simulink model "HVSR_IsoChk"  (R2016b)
settings: Solver=VariableStepAuto  StartTime=0.0  StopTime=10.0  RelTol=1e-3
undefined symbols (not defined in the file or in its folder): bin2dec, enmActv, enmBmsMode, enmCctErr, enmSWSta, HVSR_bIsoResShieldCal, HVSR_bSw1EnaByMnl_C, HVSR_bSw2EnaByMnl_C, HVSR_bSw3EnaByMnl_C, HVSR_bSwEnaByMnl_C, HVSR_bVldEnaByMnl_C, HVSR_cntIsoChkCnfDiag_C, HVSR_cntIsoChkCnfLv1Diag_C, HVSR_cntIsoChkDiag_CW, HVSR_cntPwrDown_C, HVSR_cofPosVoltfilter_C, HVSR_cofResGain_C, HVSR_deltInsRes_C, HVSR_InsResCtrlSw_C, HVSR_kSlopeVal_C, HVSR_numBgnTimeCnt_C, HVSR_numCycleTimeCnt_C, HVSR_numIsoCnst_C, HVSR_numSlopeCnfrm_C, HVSR_ResFirstCtrlSw_C, HVSR_resIsoFaultLvl1Thres_C, HVSR_resIsoFaultLvl2Thres_C, HVSR_ResR1_C, HVSR_ResR2_C, HVSR_ResR3_C, HVSR_resRstnUpLim_C, HVSR_rIsoCnfHysDiag_C, HVSR_rIsoCnfHysLv1Diag_C, HVSR_stBMSModeLvl_C, HVSR_tiChkFilteTime_C, HVSR_tiIsoChkCycl_T, HVSR_tiIsoChkDebounce_C, HVSR_tiIsoVldChkDebounce_C, HVSR_tiTaskTime_C, HVSR_tiVoltDiffThres_C, HVSR_uBattVoltRngHi_C, HVSR_uBattVoltRngLo_C, HVSR_uIsoKVoltThres_C, HVSR_uIsoPosVoltFilter_C, HVSR_uIsoVoltThres_C
libraries: simulink x78
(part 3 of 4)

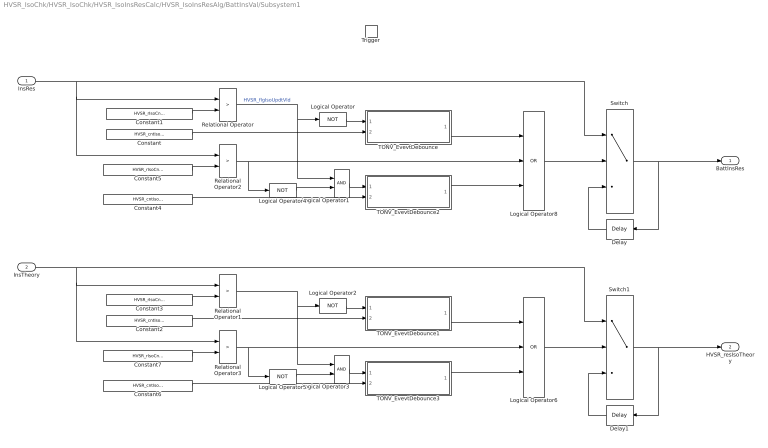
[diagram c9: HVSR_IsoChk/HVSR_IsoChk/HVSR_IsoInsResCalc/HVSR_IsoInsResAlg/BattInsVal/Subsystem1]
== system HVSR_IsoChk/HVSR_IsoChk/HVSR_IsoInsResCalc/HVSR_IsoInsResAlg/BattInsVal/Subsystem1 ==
  InsRes : Inport
  InsTheory : Inport  Port=2
  Trigger : TriggerPort  TriggerType=falling  VariantControl=Variant  PortDimensions=1
  Constant : Constant  Value=HVSR_cntIsoChkCnfDiag_C
  Constant1 : Constant  Value=HVSR_rIsoCnfHysDiag_C
  Constant2 : Constant  Value=HVSR_cntIsoChkCnfDiag_C
  Constant3 : Constant  Value=HVSR_rIsoCnfHysDiag_C
  Constant4 : Constant  Value=HVSR_cntIsoChkCnfLv1Diag_C
  Constant5 : Constant  Value=HVSR_rIsoCnfHysLv1Diag_C
  Constant6 : Constant  Value=HVSR_cntIsoChkCnfLv1Diag_C
  Constant7 : Constant  Value=HVSR_rIsoCnfHysLv1Diag_C
  Delay : Delay  DelayLength=1  InitialCondition=0
  Delay1 : Delay  DelayLength=1  InitialCondition=0
  Logical Operator{,2,4..5} (4 alike) : Logic  Operator=NOT  AllPortsSameDT=off  OutDataTypeStr=boolean
  Logical Operator1 : Logic  AllPortsSameDT=off  OutDataTypeStr=boolean
  Logical Operator3 : Logic  AllPortsSameDT=off  OutDataTypeStr=boolean
  Logical Operator6 : Logic  Operator=OR  Inputs=3  AllPortsSameDT=off  OutDataTypeStr=boolean
  Logical Operator8 : Logic  Operator=OR  Inputs=3  AllPortsSameDT=off  OutDataTypeStr=boolean
  Relational Operator{,1..3} (4 alike) : RelationalOperator  Operator=>  OutDataTypeStr=boolean  RndMeth=Simplest
  Switch : Switch  Criteria=u2 > Threshold
  Switch1 : Switch  Criteria=u2 > Threshold
  TONV_EvevtDebounce : Subsystem  TreatAsAtomicUnit=on  RTWFcnName=TONV_EvevtDebounce  RTWFileName=SrvLib
  TONV_EvevtDebounce1 : Subsystem  TreatAsAtomicUnit=on  RTWFcnName=TONV_EvevtDebounce  RTWFileName=SrvLib
  TONV_EvevtDebounce2 : Subsystem  TreatAsAtomicUnit=on  RTWFcnName=TONV_EvevtDebounce  RTWFileName=SrvLib
  TONV_EvevtDebounce3 : Subsystem  TreatAsAtomicUnit=on  RTWFcnName=TONV_EvevtDebounce  RTWFileName=SrvLib
  BattInsRes : Outport
  HVSR_resIsoTheory : Outport  Port=2
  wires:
  Constant1/1 -> Relational Operator/2
  InsRes/1 -> Relational Operator2/1, Relational Operator/1, Switch/1
  Relational Operator/1 -> Logical Operator1/1, Logical Operator/1  "HVSR_flgIsoUpdtVld"
  Switch/1 -> Delay/1, BattInsRes/1
  Logical Operator/1 -> TONV_EvevtDebounce/1(u)
  Constant/1 -> TONV_EvevtDebounce/2(T)
  Delay/1 -> Switch/3
  Constant5/1 -> Relational Operator2/2
  Logical Operator4/1 -> Logical Operator1/2
  Constant4/1 -> TONV_EvevtDebounce2/2(T)
  Relational Operator2/1 -> Logical Operator8/2, Logical Operator4/1
  TONV_EvevtDebounce2/1(y) -> Logical Operator8/3
  TONV_EvevtDebounce/1(y) -> Logical Operator8/1
  Logical Operator1/1 -> TONV_EvevtDebounce2/1(u)
  Logical Operator8/1 -> Switch/2
  Constant3/1 -> Relational Operator1/2
  InsTheory/1 -> Relational Operator3/1, Relational Operator1/1, Switch1/1
  Relational Operator1/1 -> Logical Operator3/1, Logical Operator2/1
  Switch1/1 -> HVSR_resIsoTheory/1, Delay1/1
  Logical Operator2/1 -> TONV_EvevtDebounce1/1(u)
  Constant2/1 -> TONV_EvevtDebounce1/2(T)
  Delay1/1 -> Switch1/3
  Constant7/1 -> Relational Operator3/2
  Logical Operator5/1 -> Logical Operator3/2
  Constant6/1 -> TONV_EvevtDebounce3/2(T)
  Relational Operator3/1 -> Logical Operator6/2, Logical Operator5/1
  TONV_EvevtDebounce3/1(y) -> Logical Operator6/3
  TONV_EvevtDebounce1/1(y) -> Logical Operator6/1
  Logical Operator3/1 -> TONV_EvevtDebounce3/1(u)
  Logical Operator6/1 -> Switch1/2

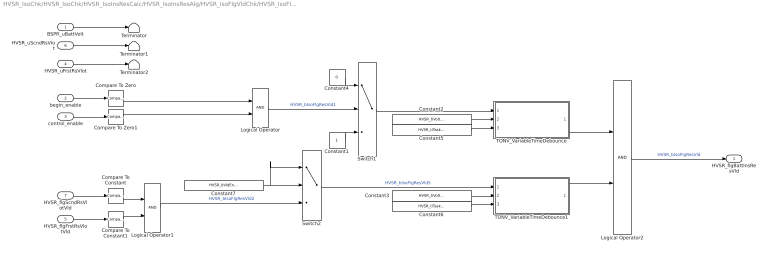
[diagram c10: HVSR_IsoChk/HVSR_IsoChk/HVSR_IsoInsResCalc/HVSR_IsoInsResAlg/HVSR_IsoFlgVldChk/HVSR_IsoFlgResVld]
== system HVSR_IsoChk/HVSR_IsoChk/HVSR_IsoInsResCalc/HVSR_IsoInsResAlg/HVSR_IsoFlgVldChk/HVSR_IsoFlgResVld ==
  BSPR_uBattVolt : Inport
  begin_enable : Inport  Port=2
  control_enable : Inport  Port=3
  HVSR_uFrstRsVlot : Inport  Port=4
  HVSR_flgFrstRsVlotVld : Inport  Port=5
  HVSR_uScndRsVlot : Inport  Port=6
  HVSR_flgScndRsVlotVld : Inport  Port=7
  Compare To Constant : simulink/Logic and Bit Operations/Compare To Constant  relop===  const=1  OutDataTypeStr=boolean
  Compare To Constant1 : simulink/Logic and Bit Operations/Compare To Constant  relop===  const=1  OutDataTypeStr=boolean
  Compare To Zero : simulink/Logic and Bit Operations/Compare To Zero  relop===  OutDataTypeStr=boolean
  Compare To Zero1 : simulink/Logic and Bit Operations/Compare To Zero  relop===  OutDataTypeStr=boolean
  Constant1 : Constant  OutDataTypeStr=boolean
  Constant2 : Constant  Value=HVSR_tiVoltDiffThres_C
  Constant3 : Constant  Value=HVSR_tiVoltDiffThres_C
  Constant4 : Constant  Value=0  OutDataTypeStr=boolean
  Constant5 : Constant  Value=HVSR_tiTaskTime_C
  Constant6 : Constant  Value=HVSR_tiTaskTime_C
  Constant7 : Constant  Value=HVSR_bVldEnaByMnl_C
  Logical Operator : Logic  AllPortsSameDT=off  OutDataTypeStr=boolean
  Logical Operator1 : Logic  AllPortsSameDT=off  OutDataTypeStr=boolean
  Logical Operator2 : Logic  AllPortsSameDT=off  OutDataTypeStr=boolean
  Switch1 : Switch  Criteria=u2 > Threshold
  Switch2 : Switch  Criteria=u2 ~= 0
  TONV_VariableTimeDebounce : Subsystem  TreatAsAtomicUnit=on  RTWFcnName=TONV_VariableTimeDebounce  RTWFileName=SrvLib
  TONV_VariableTimeDebounce1 : Subsystem  TreatAsAtomicUnit=on  RTWFcnName=TONV_VariableTimeDebounce  RTWFileName=SrvLib
  Terminator : Terminator
  Terminator1 : Terminator
  Terminator2 : Terminator
  HVSR_flgBattInsResVld : Outport
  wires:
  Constant4/1 -> Switch1/1
  Logical Operator/1 -> Switch1/2  "HVSR_bIsoFlgResVld1"
  Compare To Zero1/1 -> Logical Operator/2
  Compare To Zero/1 -> Logical Operator/1
  control_enable/1 -> Compare To Zero1/1
  begin_enable/1 -> Compare To Zero/1
  Logical Operator2/1 -> HVSR_flgBattInsResVld/1  "HVSR_bIsoFlgResVld"
  Constant3/1 -> TONV_VariableTimeDebounce1/2(T)
  Constant6/1 -> TONV_VariableTimeDebounce1/3(dT)
  TONV_VariableTimeDebounce1/1(y) -> Logical Operator2/2
  Constant2/1 -> TONV_VariableTimeDebounce/2(T)
  Constant5/1 -> TONV_VariableTimeDebounce/3(dT)
  Switch1/1 -> TONV_VariableTimeDebounce/1(u)
  TONV_VariableTimeDebounce/1(y) -> Logical Operator2/1
  BSPR_uBattVolt/1 -> Terminator/1
  HVSR_uScndRsVlot/1 -> Terminator1/1
  HVSR_uFrstRsVlot/1 -> Terminator2/1
  HVSR_flgScndRsVlotVld/1 -> Compare To Constant/1
  HVSR_flgFrstRsVlotVld/1 -> Compare To Constant1/1
  Logical Operator1/1 -> Switch2/3  "HVSR_bIsoFlgResVld2"
  Constant1/1 -> Switch1/3
  Constant7/1 -> Switch2/1, Switch2/2
  Switch2/1 -> TONV_VariableTimeDebounce1/1(u)  "HVSR_bIsoFlgResVld5"
  Compare To Constant/1 -> Logical Operator1/1
  Compare To Constant1/1 -> Logical Operator1/2

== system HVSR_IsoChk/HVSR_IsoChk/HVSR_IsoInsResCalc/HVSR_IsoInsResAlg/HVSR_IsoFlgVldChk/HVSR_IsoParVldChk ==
  HVSR_flgBattInsResVld : Inport
  HVSR_uFrstRsVlot : Inport  Port=2
  HVSR_flgFrstRsVlotVld : Inport  Port=3
  HVSR_uScndRsVlot : Inport  Port=4
  HVSR_flgScndRsVlotVld : Inport  Port=5
  In6 : Inport  Port=6
  IsoSwtLastTEna : Inport  Port=7
  Compare To Zero{,1..3} (4 alike) : simulink/Logic and Bit Operations/Compare To Zero  relop=~=  OutDataTypeStr=boolean
  Constant : Constant  Value=0  OutDataTypeStr=boolean
  Logical Operator : Logic  Inputs=6  AllPortsSameDT=off  OutDataTypeStr=boolean
  Switch : Switch  Criteria=u2 ~= 0
  HVSR_flgInsResVld : Outport
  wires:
  Switch/1 -> HVSR_flgInsResVld/1
  Compare To Zero3/1 -> Logical Operator/4
  Compare To Zero2/1 -> Logical Operator/3
  Compare To Zero1/1 -> Logical Operator/2
  Compare To Zero/1 -> Logical Operator/1
  HVSR_flgBattInsResVld/1 -> Switch/1
  Constant/1 -> Switch/3
  Logical Operator/1 -> Switch/2  "HVSR_bIsoFlgResVld3"
  IsoSwtLastTEna/1 -> Logical Operator/6
  HVSR_uScndRsVlot/1 -> Compare To Zero2/1
  HVSR_flgScndRsVlotVld/1 -> Compare To Zero3/1
  HVSR_uFrstRsVlot/1 -> Compare To Zero/1
  HVSR_flgFrstRsVlotVld/1 -> Compare To Zero1/1
  In6/1 -> Logical Operator/5

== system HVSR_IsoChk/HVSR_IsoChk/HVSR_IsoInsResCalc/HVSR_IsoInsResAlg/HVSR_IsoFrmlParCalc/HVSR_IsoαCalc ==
  HVSR_uIsoRsVolt : Inport  OutDataTypeStr=single
  HVSR_kSlopeVal : Inport  Port=2  OutDataTypeStr=single
  HVSR_tiIsoChkCycl_T : Inport  Port=3  OutDataTypeStr=single
  HVSR_numSlopeCnfrm : Inport  Port=4
  BSPR_uBattVolt : Inport  Port=5
  Action Port : ActionPort  InitializeStates=reset  ActionType=then
  HVSR_IsoαParCalc : Subsystem
  HVSR_uRsFrstSlopeFilter : Subsystem
  HVSR_uRsVoltFilter : Subsystem
  Logical Operator : Logic  AllPortsSameDT=off  OutDataTypeStr=boolean
  Terminator : Terminator
  HVSR_uIsoFrstRsVolt : Outport  InitialOutput=0
  HVSR_uFrstRsVlot : Outport  Port=2  InitialOutput=0
  HVSR_flgFrstRsVlotVld : Outport  Port=3
  HVSR_numIsoFrstVal : Outport  Port=4
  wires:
  HVSR_uRsVoltFilter/1(HVSR_uIsoFrstRsVolt) -> HVSR_uIsoFrstRsVolt/1
  BSPR_uBattVolt/1 -> HVSR_IsoαParCalc/2(BSPR_uBattVolt)
  HVSR_uRsVoltFilter/3(HVSR_flgFrstRsKVld) -> Logical Operator/1  "HVSR_flgFrstRsKVld"
  HVSR_IsoαParCalc/1(HVSR_numIsoFrstVal) -> HVSR_numIsoFrstVal/1
  HVSR_uIsoRsVolt/1 -> HVSR_uRsFrstSlopeFilter/1(HVSR_uIsoRsVolt), HVSR_uRsVoltFilter/1(HVSR_uIsoRsVolt)
  HVSR_uRsVoltFilter/2(HVSR_uFrstRsVlot) -> HVSR_uFrstRsVlot/1, [HVSR_uFrstRsVlot]
  Logical Operator/1 -> HVSR_flgFrstRsVlotVld/1, HVSR_IsoαParCalc/Trigger  "HVSR_flgFrstRsVlotVld"
  [HVSR_uFrstRsVlot] -> HVSR_IsoαParCalc/1(HVSR_uFrstRsVlot)
  HVSR_kSlopeVal/1 -> HVSR_uRsFrstSlopeFilter/2(HVSR_kSlopeVal)
  HVSR_tiIsoChkCycl_T/1 -> HVSR_uRsFrstSlopeFilter/3(HVSR_tiIsoChkCycl_T)
  HVSR_numSlopeCnfrm/1 -> HVSR_uRsFrstSlopeFilter/4(HVSR_numSlopeCnfrm)
  HVSR_uRsFrstSlopeFilter/1(HVSR_bSlopeVld) -> Logical Operator/2  "HVSR_bFrstSlopeVld"
  HVSR_uRsFrstSlopeFilter/2(ISOFilterSta) -> Terminator/1

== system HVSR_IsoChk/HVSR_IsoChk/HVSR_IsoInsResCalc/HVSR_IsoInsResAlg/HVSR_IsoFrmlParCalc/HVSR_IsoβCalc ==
  HVSR_uIsoRsVolt : Inport  OutDataTypeStr=single
  HVSR_kSlopeVal : Inport  Port=2  OutDataTypeStr=single
  HVSR_tiIsoChkCycl_T : Inport  Port=3  OutDataTypeStr=single
  HVSR_numSlopeCnfrm : Inport  Port=4  OutDataTypeStr=uint8
  BSPR_uBattVolt : Inport  Port=5
  Action Port : ActionPort  InitializeStates=reset  ActionType=elseif
  HVSR_IsoβParCalc : Subsystem
  HVSR_uRsScndSlopeFilter : Subsystem
  HVSR_uRsVoltFilter : Subsystem
  Logical Operator : Logic  AllPortsSameDT=off  OutDataTypeStr=boolean
  Terminator : Terminator
  HVSR_uIsoScndRsVolt : Outport  InitialOutput=0
  HVSR_uScndRsVlot : Outport  Port=2  InitialOutput=0
  HVSR_flgScndRsVlotVld : Outport  Port=3
  HVSR_numIsoScndVal : Outport  Port=4
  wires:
  HVSR_uRsVoltFilter/1(HVSR_uIsoScndRsVolt) -> HVSR_uIsoScndRsVolt/1
  HVSR_uIsoRsVolt/1 -> HVSR_uRsScndSlopeFilter/1(HVSR_uIsoRsVolt), HVSR_uRsVoltFilter/1(HVSR_uIsoRsVolt)
  HVSR_uRsVoltFilter/2(HVSR_uScndRsVlot) -> HVSR_uScndRsVlot/1, [HVSR_uScndRsVlot]
  BSPR_uBattVolt/1 -> HVSR_IsoβParCalc/2(BSPR_uBattVolt)
  HVSR_uRsVoltFilter/3(HVSR_flgScndRsKVld) -> Logical Operator/1  "HVSR_flgScndRsKVld"
  HVSR_IsoβParCalc/1(HVSR_numIsoScndVal) -> HVSR_numIsoScndVal/1
  HVSR_kSlopeVal/1 -> HVSR_uRsScndSlopeFilter/2(HVSR_kSlopeVal)
  HVSR_tiIsoChkCycl_T/1 -> HVSR_uRsScndSlopeFilter/3(HVSR_tiIsoChkCycl_T)
  HVSR_numSlopeCnfrm/1 -> HVSR_uRsScndSlopeFilter/4(HVSR_numSlopeCnfrm)
  HVSR_uRsScndSlopeFilter/1(HVSR_bSlopeVld) -> Logical Operator/2  "HVSR_bScndSlopeVld"
  HVSR_uRsScndSlopeFilter/2(ISOFilterSta) -> Terminator/1
  Logical Operator/1 -> HVSR_flgScndRsVlotVld/1, HVSR_IsoβParCalc/Trigger  "HVSR_flgScndRsVlotVld"
  [HVSR_uScndRsVlot] -> HVSR_IsoβParCalc/1(HVSR_uScndRsVlot)

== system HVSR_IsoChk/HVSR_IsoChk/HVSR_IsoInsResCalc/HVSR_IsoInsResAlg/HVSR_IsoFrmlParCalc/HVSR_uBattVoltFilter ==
  BSPR_uBattVolt : Inport  OutDataTypeStr=single
  Compare To Constant : simulink/Logic and Bit Operations/Compare To Constant  relop=<=  const=HVSR_uIsoVoltThres_C  OutDataTypeStr=boolean
  Constant2 : Constant  Value=0  OutDataTypeStr=single
  Subsystem2 : Subsystem
  Switch : Switch  Criteria=u2 > Threshold
  HVSR_uBattVolt : Outport
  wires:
  Constant2/1 -> Switch/3
  Switch/1 -> HVSR_uBattVolt/1
  Compare To Constant/1 -> Switch/2  "HVSR_flgBattFilterEnd"
  Subsystem2/1(Out1) -> Compare To Constant/1  "HVSR_uBattFltDiff"
  BSPR_uBattVolt/1 -> Subsystem2/1(In1), Switch/1

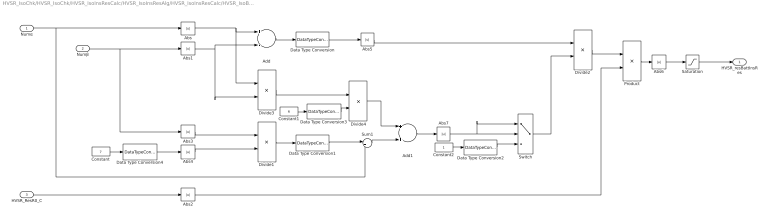
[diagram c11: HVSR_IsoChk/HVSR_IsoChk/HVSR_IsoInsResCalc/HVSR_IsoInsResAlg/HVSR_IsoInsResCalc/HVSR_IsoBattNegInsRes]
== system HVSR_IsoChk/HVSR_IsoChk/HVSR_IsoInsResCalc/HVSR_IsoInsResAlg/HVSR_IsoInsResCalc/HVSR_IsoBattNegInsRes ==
  Numα : Inport
  Numβ : Inport  Port=2
  HVSR_ResR0_C : Inport  Port=3
  Abs{,1..7} (8 alike) : Abs
  Add : Sum  Inputs=+-
  Add1 : Sum
  Constant : Constant  Value=7
  Constant1 : Constant  Value=6
  Constant2 : Constant
  Data Type Conversion : DataTypeConversion
  Data Type Conversion1 : DataTypeConversion
  Data Type Conversion2 : DataTypeConversion  OutDataTypeStr=single
  Data Type Conversion3 : DataTypeConversion  OutDataTypeStr=single
  Data Type Conversion4 : DataTypeConversion  OutDataTypeStr=single
  Divide1 : Product  Inputs=**
  Divide2 : Product  Inputs=*/
  Divide3 : Product  Inputs=**
  Divide4 : Product  Inputs=**
  Product : Product
  Saturation : Saturate  UpperLimit=60000000  LowerLimit=0
  Sum1 : Sum  Inputs=|+-
  Switch : Switch  Criteria=u2 > Threshold
  HVSR_resBattInsRes : Outport
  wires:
  Switch/1 -> Divide2/2
  Data Type Conversion2/1 -> Switch/3
  Constant2/1 -> Data Type Conversion2/1
  Divide2/1 -> Product/1
  Abs7/1 -> Switch/2, Switch/1
  Add1/1 -> Abs7/1
  Data Type Conversion/1 -> Abs5/1
  Data Type Conversion3/1 -> Divide4/2
  Constant1/1 -> Data Type Conversion3/1
  Sum1/1 -> Add1/2
  Data Type Conversion1/1 -> Sum1/1
  Data Type Conversion4/1 -> Abs4/1
  Constant/1 -> Data Type Conversion4/1
  HVSR_ResR0_C/1 -> Abs2/1
  Numβ/1 -> Abs3/1, Abs1/1
  Numα/1 -> Sum1/2, Abs/1
  Abs1/1 -> Divide3/2, Add/2
  Abs3/1 -> Divide1/1
  Abs2/1 -> Product/2
  Abs4/1 -> Divide1/2
  Abs/1 -> Divide3/1, Add/1
  Divide1/1 -> Data Type Conversion1/1
  Abs5/1 -> Divide2/1
  Add/1 -> Data Type Conversion/1
  Abs6/1 -> Saturation/1
  Product/1 -> Abs6/1
  Saturation/1 -> HVSR_resBattInsRes/1
  Divide3/1 -> Divide4/1
  Divide4/1 -> Add1/1

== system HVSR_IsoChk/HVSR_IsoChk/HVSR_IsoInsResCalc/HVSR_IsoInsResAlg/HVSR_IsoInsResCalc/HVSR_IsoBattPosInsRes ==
  Numα : Inport
  Numβ : Inport  Port=2
  HVSR_ResR0_C : Inport  Port=3
  Abs{,1..7} (8 alike) : Abs
  Add : Sum  Inputs=+-
  Add1 : Sum
  Constant : Constant  Value=7
  Constant1 : Constant  Value=6
  Constant2 : Constant
  Data Type Conversion : DataTypeConversion
  Data Type Conversion1 : DataTypeConversion
  Data Type Conversion2 : DataTypeConversion  OutDataTypeStr=single
  Data Type Conversion3 : DataTypeConversion  OutDataTypeStr=single
  Data Type Conversion4 : DataTypeConversion  OutDataTypeStr=single
  Divide1 : Product  Inputs=**
  Divide2 : Product  Inputs=*/
  Product : Product
  Saturation : Saturate  UpperLimit=60000000  LowerLimit=0
  Sum1 : Sum  Inputs=|+-
  Switch : Switch  Criteria=u2 > Threshold
  HVSR_resBattInsRes : Outport
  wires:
  Saturation/1 -> HVSR_resBattInsRes/1
  Product/1 -> Abs6/1
  Abs6/1 -> Saturation/1
  Add/1 -> Data Type Conversion/1
  Abs5/1 -> Divide2/1
  Divide1/1 -> Data Type Conversion1/1
  Abs/1 -> Add/1
  Abs4/1 -> Divide1/2
  Abs2/1 -> Product/2
  Abs3/1 -> Divide1/1
  Abs1/1 -> Add/2
  Numα/1 -> Abs/1, Sum1/2
  Numβ/1 -> Abs1/1, Abs3/1
  HVSR_ResR0_C/1 -> Abs2/1
  Constant/1 -> Data Type Conversion4/1
  Data Type Conversion4/1 -> Abs4/1
  Data Type Conversion1/1 -> Sum1/1
  Sum1/1 -> Add1/2
  Constant1/1 -> Data Type Conversion3/1
  Data Type Conversion3/1 -> Add1/1
  Data Type Conversion/1 -> Abs5/1
  Add1/1 -> Abs7/1
  Abs7/1 -> Switch/1, Switch/2
  Divide2/1 -> Product/1
  Constant2/1 -> Data Type Conversion2/1
  Data Type Conversion2/1 -> Switch/3
  Switch/1 -> Divide2/2

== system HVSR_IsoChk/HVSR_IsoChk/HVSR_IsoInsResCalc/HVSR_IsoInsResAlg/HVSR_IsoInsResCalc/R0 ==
  Constant1 : Constant  Value=HVSR_numIsoCnst_C
  Data Type Conversion1 : DataTypeConversion  OutDataTypeStr=single
  HVSR_ResR0_C : Outport
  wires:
  Constant1/1 -> Data Type Conversion1/1
  Data Type Conversion1/1 -> HVSR_ResR0_C/1

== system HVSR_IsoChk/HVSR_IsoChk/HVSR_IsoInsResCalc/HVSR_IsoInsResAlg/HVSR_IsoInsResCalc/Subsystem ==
  Rp' : Inport
  Abs : Abs
  Constant1 : Constant  Value=HVSR_ResR1_C  OutDataTypeStr=single
  Constant2 : Constant  Value=HVSR_ResR2_C  OutDataTypeStr=single
  Constant3 : Constant  Value=HVSR_ResR3_C  OutDataTypeStr=single
  Data Type Conversion : DataTypeConversion  OutDataTypeStr=single
  Data Type Conversion1 : DataTypeConversion  OutDataTypeStr=single
  Divide : Product  Inputs=/*  OutDataTypeStr=double
  Product : Product  OutDataTypeStr=double
  Saturation : Saturate  UpperLimit=60000000  LowerLimit=0
  Sum : Sum  Inputs=|++
  Sum1 : Sum  Inputs=|++
  Sum2 : Sum  Inputs=|-+
  HVSR_resIsoTheory : Outport
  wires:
  Saturation/1 -> HVSR_resIsoTheory/1
  Abs/1 -> Saturation/1
  Data Type Conversion1/1 -> Divide/2
  Product/1 -> Data Type Conversion1/1
  Data Type Conversion/1 -> Abs/1
  Divide/1 -> Data Type Conversion/1
  Sum2/1 -> Divide/1
  Rp'/1 -> Product/1, Sum2/1
  Sum1/1 -> Product/2, Sum2/2
  Constant2/1 -> Sum1/2
  Sum/1 -> Sum1/1
  Constant3/1 -> Sum/2
  Constant1/1 -> Sum/1

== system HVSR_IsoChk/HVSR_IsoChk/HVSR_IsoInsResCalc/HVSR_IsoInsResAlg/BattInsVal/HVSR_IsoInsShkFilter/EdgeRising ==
  u : Inport
  Delay1 : Delay  DelayLength=1  InitialCondition=1
  Logical Operator3 : Logic  Operator=NOT  AllPortsSameDT=off  OutDataTypeStr=boolean
  Logical Operator4 : Logic  AllPortsSameDT=off  OutDataTypeStr=boolean
  y : Outport
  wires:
  Delay1/1 -> Logical Operator3/1
  u/1 -> Logical Operator4/2, Delay1/1
  Logical Operator3/1 -> Logical Operator4/1
  Logical Operator4/1 -> y/1

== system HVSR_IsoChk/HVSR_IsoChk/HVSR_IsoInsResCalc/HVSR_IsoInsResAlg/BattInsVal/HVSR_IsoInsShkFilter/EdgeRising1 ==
  u : Inport
  Delay1 : Delay  DelayLength=1  InitialCondition=1
  Logical Operator3 : Logic  Operator=NOT  AllPortsSameDT=off  OutDataTypeStr=boolean
  Logical Operator4 : Logic  AllPortsSameDT=off  OutDataTypeStr=boolean
  y : Outport
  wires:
  Logical Operator4/1 -> y/1
  Logical Operator3/1 -> Logical Operator4/1
  u/1 -> Delay1/1, Logical Operator4/2
  Delay1/1 -> Logical Operator3/1

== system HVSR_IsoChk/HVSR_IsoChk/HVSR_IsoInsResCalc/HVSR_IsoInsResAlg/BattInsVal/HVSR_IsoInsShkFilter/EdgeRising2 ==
  u : Inport
  Delay1 : Delay  DelayLength=1  InitialCondition=1
  Logical Operator3 : Logic  Operator=NOT  AllPortsSameDT=off  OutDataTypeStr=boolean
  Logical Operator4 : Logic  AllPortsSameDT=off  OutDataTypeStr=boolean
  y : Outport
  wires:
  Delay1/1 -> Logical Operator3/1
  u/1 -> Logical Operator4/2, Delay1/1
  Logical Operator3/1 -> Logical Operator4/1
  Logical Operator4/1 -> y/1

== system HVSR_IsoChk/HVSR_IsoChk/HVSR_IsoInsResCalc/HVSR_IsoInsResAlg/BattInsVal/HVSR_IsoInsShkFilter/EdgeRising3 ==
  u : Inport
  Delay1 : Delay  DelayLength=1  InitialCondition=1
  Logical Operator3 : Logic  Operator=NOT  AllPortsSameDT=off  OutDataTypeStr=boolean
  Logical Operator4 : Logic  AllPortsSameDT=off  OutDataTypeStr=boolean
  y : Outport
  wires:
  Logical Operator4/1 -> y/1
  Logical Operator3/1 -> Logical Operator4/1
  u/1 -> Delay1/1, Logical Operator4/2
  Delay1/1 -> Logical Operator3/1

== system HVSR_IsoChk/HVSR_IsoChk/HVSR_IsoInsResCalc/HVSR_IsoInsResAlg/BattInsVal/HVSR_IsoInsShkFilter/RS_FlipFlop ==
  S : Inport  OutDataTypeStr=boolean
  R : Inport  Port=2  OutDataTypeStr=boolean
  RS : Stateflow chart  TreatAsAtomicUnit=on
  Q : Outport  OutDataTypeStr=boolean
  !Q : Outport  Port=2  OutDataTypeStr=boolean
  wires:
  R/1 -> RS/2(R)
  S/1 -> RS/1(S)
  RS/2(nQ) -> !Q/1
  RS/1(Q) -> Q/1

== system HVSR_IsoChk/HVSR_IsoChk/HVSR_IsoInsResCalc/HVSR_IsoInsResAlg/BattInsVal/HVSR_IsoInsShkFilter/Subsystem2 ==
  In1 : Inport
  Enable : EnablePort
  Out1 : Outport
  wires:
  In1/1 -> Out1/1

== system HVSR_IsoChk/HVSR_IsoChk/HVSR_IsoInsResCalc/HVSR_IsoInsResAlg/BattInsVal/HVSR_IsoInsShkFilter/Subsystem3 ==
  set : Inport
  clear : Inport  Port=2
  Delay : Delay  DelayLength=1  InitialCondition=0
  Logical Operator : Logic  Operator=OR  AllPortsSameDT=off  OutDataTypeStr=boolean
  Logical Operator4 : Logic  AllPortsSameDT=off  OutDataTypeStr=boolean
  Logical Operator5 : Logic  Operator=NOT  AllPortsSameDT=off  OutDataTypeStr=boolean
  Q : Outport
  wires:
  Delay/1 -> Logical Operator/1
  Logical Operator4/1 -> Q/1, Delay/1
  Logical Operator/1 -> Logical Operator4/1
  Logical Operator5/1 -> Logical Operator4/2
  clear/1 -> Logical Operator5/1
  set/1 -> Logical Operator/2

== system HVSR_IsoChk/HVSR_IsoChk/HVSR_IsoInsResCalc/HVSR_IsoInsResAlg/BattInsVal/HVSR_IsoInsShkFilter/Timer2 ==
  En : Inport
  Ts : Inport  Port=2
  Rst : Inport  Port=3
  Vst : Inport  Port=4
  Add : Sum
  Constant5 : Constant  Value=single(0)  OutDataTypeStr=single
  Switch1 : Switch  Criteria=u2 ~= 0
  Switch2 : Switch  Criteria=u2 ~= 0
  Unit Delay : UnitDelay  SampleTime=-1
  Timer : Outport
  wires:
  Unit Delay/1 -> Add/2
  Rst/1 -> Switch1/2
  En/1 -> Switch2/2
  Ts/1 -> Switch2/1
  Constant5/1 -> Switch2/3
  Switch2/1 -> Add/1
  Vst/1 -> Switch1/1
  Switch1/1 -> Timer/1, Unit Delay/1
  Add/1 -> Switch1/3

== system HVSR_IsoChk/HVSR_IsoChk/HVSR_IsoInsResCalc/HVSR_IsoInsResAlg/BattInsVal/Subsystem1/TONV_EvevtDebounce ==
  note: Turn On Delay Evevt Deboune
  u : Inport
  T : Inport  Port=2
  Add : Sum
  Constant : Constant  OutDataTypeStr=uint8
  Constant1 : Constant  Value=0  OutDataTypeStr=uint8
  Delay : Delay  DelayLength=1  InitialCondition=0
  MinMax : MinMax  Inputs=2
  Product : Product  OutMin=[0]  OutMax=[65535]  OutDataTypeStr=single
  Relational Operator : RelationalOperator  Operator=>  OutDataTypeStr=boolean  RndMeth=Simplest
  Switch : Switch  Criteria=u2 > Threshold
  y : Outport
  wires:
  MinMax/1 -> Add/2
  T/1 -> MinMax/1, Relational Operator/2
  Relational Operator/1 -> y/1
  Delay/1 -> MinMax/2
  Switch/1 -> Product/1, Add/1
  Product/1 -> Delay/1, Relational Operator/1
  Add/1 -> Product/2
  Constant1/1 -> Switch/3
  Constant/1 -> Switch/1
  u/1 -> Switch/2

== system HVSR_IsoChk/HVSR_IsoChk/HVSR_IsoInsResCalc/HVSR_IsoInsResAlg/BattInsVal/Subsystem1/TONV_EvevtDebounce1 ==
  note: Turn On Delay Evevt Deboune
  u : Inport
  T : Inport  Port=2
  Add : Sum
  Constant : Constant  OutDataTypeStr=uint8
  Constant1 : Constant  Value=0  OutDataTypeStr=uint8
  Delay : Delay  DelayLength=1  InitialCondition=0
  MinMax : MinMax  Inputs=2
  Product : Product  OutMin=[0]  OutMax=[65535]  OutDataTypeStr=single
  Relational Operator : RelationalOperator  Operator=>  OutDataTypeStr=boolean  RndMeth=Simplest
  Switch : Switch  Criteria=u2 > Threshold
  y : Outport
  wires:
  MinMax/1 -> Add/2
  T/1 -> MinMax/1, Relational Operator/2
  Relational Operator/1 -> y/1
  Delay/1 -> MinMax/2
  Switch/1 -> Product/1, Add/1
  Product/1 -> Delay/1, Relational Operator/1
  Add/1 -> Product/2
  Constant1/1 -> Switch/3
  Constant/1 -> Switch/1
  u/1 -> Switch/2

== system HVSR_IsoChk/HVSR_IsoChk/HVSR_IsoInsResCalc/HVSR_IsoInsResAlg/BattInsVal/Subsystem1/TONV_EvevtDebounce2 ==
  note: Turn On Delay Evevt Deboune
  u : Inport
  T : Inport  Port=2
  Add : Sum
  Constant : Constant  OutDataTypeStr=uint8
  Constant1 : Constant  Value=0  OutDataTypeStr=uint8
  Delay : Delay  DelayLength=1  InitialCondition=0
  MinMax : MinMax  Inputs=2
  Product : Product  OutMin=[0]  OutMax=[65535]  OutDataTypeStr=single
  Relational Operator : RelationalOperator  Operator=>  OutDataTypeStr=boolean  RndMeth=Simplest
  Switch : Switch  Criteria=u2 > Threshold
  y : Outport
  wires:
  u/1 -> Switch/2
  Constant/1 -> Switch/1
  Constant1/1 -> Switch/3
  Add/1 -> Product/2
  Product/1 -> Relational Operator/1, Delay/1
  Switch/1 -> Add/1, Product/1
  Delay/1 -> MinMax/2
  Relational Operator/1 -> y/1
  T/1 -> Relational Operator/2, MinMax/1
  MinMax/1 -> Add/2

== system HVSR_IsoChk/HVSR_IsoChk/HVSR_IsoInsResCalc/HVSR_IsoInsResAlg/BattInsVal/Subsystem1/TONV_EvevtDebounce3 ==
  note: Turn On Delay Evevt Deboune
  u : Inport
  T : Inport  Port=2
  Add : Sum
  Constant : Constant  OutDataTypeStr=uint8
  Constant1 : Constant  Value=0  OutDataTypeStr=uint8
  Delay : Delay  DelayLength=1  InitialCondition=0
  MinMax : MinMax  Inputs=2
  Product : Product  OutMin=[0]  OutMax=[65535]  OutDataTypeStr=single
  Relational Operator : RelationalOperator  Operator=>  OutDataTypeStr=boolean  RndMeth=Simplest
  Switch : Switch  Criteria=u2 > Threshold
  y : Outport
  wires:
  u/1 -> Switch/2
  Constant/1 -> Switch/1
  Constant1/1 -> Switch/3
  Add/1 -> Product/2
  Product/1 -> Relational Operator/1, Delay/1
  Switch/1 -> Add/1, Product/1
  Delay/1 -> MinMax/2
  Relational Operator/1 -> y/1
  T/1 -> Relational Operator/2, MinMax/1
  MinMax/1 -> Add/2

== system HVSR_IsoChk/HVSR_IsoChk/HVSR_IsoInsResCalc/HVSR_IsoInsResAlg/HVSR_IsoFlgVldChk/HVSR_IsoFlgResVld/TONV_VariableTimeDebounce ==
  note: Turn On Delay Time Deboune
  u : Inport
  T : Inport  Port=2
  dT : Inport  Port=3
  Add : Sum
  Constant1 : Constant  Value=0  OutDataTypeStr=single
  Constant2 : Constant  OutDataTypeStr=uint8
  Constant3 : Constant  Value=0  OutDataTypeStr=uint8
  Delay : Delay  DelayLength=1  InitialCondition=0
  MinMax : MinMax  Inputs=2
  Product : Product  OutMin=[0]  OutMax=[65535]  OutDataTypeStr=single
  Relational Operator : RelationalOperator  Operator=>  OutDataTypeStr=boolean  RndMeth=Simplest
  Switch : Switch  Criteria=u2 ~= 0
  Switch1 : Switch  Criteria=u2 ~= 0
  y : Outport
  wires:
  Switch1/1 -> Product/1
  Constant3/1 -> Switch1/3
  Constant2/1 -> Switch1/1
  u/1 -> Switch1/2, Switch/2
  dT/1 -> Switch/1
  Constant1/1 -> Switch/3
  Add/1 -> Product/2
  Product/1 -> Relational Operator/1, Delay/1
  Switch/1 -> Add/1
  Delay/1 -> MinMax/2
  Relational Operator/1 -> y/1
  T/1 -> MinMax/1, Relational Operator/2
  MinMax/1 -> Add/2

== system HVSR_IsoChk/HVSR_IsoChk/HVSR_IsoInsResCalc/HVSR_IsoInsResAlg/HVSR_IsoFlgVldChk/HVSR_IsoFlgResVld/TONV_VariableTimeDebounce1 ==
  note: Turn On Delay Time Deboune
  u : Inport
  T : Inport  Port=2
  dT : Inport  Port=3
  Add : Sum
  Constant1 : Constant  Value=0  OutDataTypeStr=single
  Constant2 : Constant  OutDataTypeStr=uint8
  Constant3 : Constant  Value=0  OutDataTypeStr=uint8
  Delay : Delay  DelayLength=1  InitialCondition=0
  MinMax : MinMax  Inputs=2
  Product : Product  OutMin=[0]  OutMax=[65535]  OutDataTypeStr=single
  Relational Operator : RelationalOperator  Operator=>  OutDataTypeStr=boolean  RndMeth=Simplest
  Switch : Switch  Criteria=u2 ~= 0
  Switch1 : Switch  Criteria=u2 ~= 0
  y : Outport
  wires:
  MinMax/1 -> Add/2
  T/1 -> Relational Operator/2, MinMax/1
  Relational Operator/1 -> y/1
  Delay/1 -> MinMax/2
  Switch/1 -> Add/1
  Product/1 -> Delay/1, Relational Operator/1
  Add/1 -> Product/2
  Constant1/1 -> Switch/3
  dT/1 -> Switch/1
  u/1 -> Switch/2, Switch1/2
  Constant2/1 -> Switch1/1
  Constant3/1 -> Switch1/3
  Switch1/1 -> Product/1

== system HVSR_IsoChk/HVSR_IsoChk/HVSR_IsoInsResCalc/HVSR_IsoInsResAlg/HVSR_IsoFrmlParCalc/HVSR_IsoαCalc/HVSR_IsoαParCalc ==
  HVSR_uFrstRsVlot : Inport
  BSPR_uBattVolt : Inport  Port=2
  Trigger : TriggerPort  VariantControl=Variant  PortDimensions=1
  Add : Sum  Inputs=+-
  Compare To Zero : simulink/Logic and Bit Operations/Compare To Zero  relop=>  OutDataTypeStr=boolean
  Divide : Product  Inputs=*/
  Switch : Switch  Criteria=u2 ~= 0
  HVSR_numIsoFrstVal : Outport
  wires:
  BSPR_uBattVolt/1 -> Add/1, Switch/3
  Add/1 -> Divide/1
  Divide/1 -> HVSR_numIsoFrstVal/1
  Switch/1 -> Divide/2
  Compare To Zero/1 -> Switch/2
  HVSR_uFrstRsVlot/1 -> Add/2, Switch/1, Compare To Zero/1

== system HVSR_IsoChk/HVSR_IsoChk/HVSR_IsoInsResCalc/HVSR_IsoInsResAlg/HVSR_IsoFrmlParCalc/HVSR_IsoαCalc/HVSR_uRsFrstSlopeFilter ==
  HVSR_uIsoRsVolt : Inport  OutDataTypeStr=single
  HVSR_kSlopeVal : Inport  Port=2
  HVSR_tiIsoChkCycl_T : Inport  Port=3
  HVSR_numSlopeCnfrm : Inport  Port=4
  Chart : Stateflow chart  TreatAsAtomicUnit=on
  HVSR_bSlopeVld : Outport  OutDataTypeStr=boolean
  ISOFilterSta : Outport  Port=2  OutDataTypeStr=uint8
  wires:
  HVSR_numSlopeCnfrm/1 -> Chart/4(HVSR_numSlopeCnfrm)
  HVSR_tiIsoChkCycl_T/1 -> Chart/3(HVSR_tiIsoChkCycl_T)
  Chart/2(ISOFilterSta) -> ISOFilterSta/1
  HVSR_kSlopeVal/1 -> Chart/2(HVSR_kSlopeVal)
  Chart/1(HVSR_bSlopeVld) -> HVSR_bSlopeVld/1
  HVSR_uIsoRsVolt/1 -> Chart/1(HVSR_uIsoRsVolt)

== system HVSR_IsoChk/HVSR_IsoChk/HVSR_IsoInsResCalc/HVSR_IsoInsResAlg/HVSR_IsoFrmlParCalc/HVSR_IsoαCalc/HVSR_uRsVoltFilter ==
  HVSR_uIsoRsVolt : Inport  OutDataTypeStr=single
  Abs : Abs
  Constant1 : Constant  Value=HVSR_tiTaskTime_C  OutDataTypeStr=single
  Constant2 : Constant  Value=HVSR_cofPosVoltfilter_C  OutDataTypeStr=single
  Constant3 : Constant  Value=0  OutDataTypeStr=single
  Constant4 : Constant  Value=HVSR_uIsoKVoltThres_C  OutDataTypeStr=single
  Constant8 : Constant  Value=HVSR_tiChkFilteTime_C  OutDataTypeStr=single
  K_Lowpass : Subsystem  TreatAsAtomicUnit=on  RTWFcnName=K_Lowpass  RTWFileName=SrvLib
  Relational Operator1 : RelationalOperator  Operator=<=  OutDataTypeStr=boolean  RndMeth=Simplest
  Subtract : Sum  Inputs=+-
  Switch3 : Switch  Criteria=u2 ~= 0
  TONV_VariableTimeDebounce : Subsystem  TreatAsAtomicUnit=on  RTWFcnName=TONV_VariableTimeDebounce  RTWFileName=SrvLib
  HVSR_uIsoFrstRsVolt : Outport
  HVSR_uFrstRsVlot : Outport  Port=2
  HVSR_flgFrstRsKVld : Outport  Port=3
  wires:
  Switch3/1 -> HVSR_uFrstRsVlot/1
  HVSR_uIsoRsVolt/1 -> Subtract/2, Switch3/1, HVSR_uIsoFrstRsVolt/1, K_Lowpass/2(u)
  Constant3/1 -> Switch3/3
  Constant2/1 -> K_Lowpass/1(k)
  K_Lowpass/1(y) -> Subtract/1
  Subtract/1 -> Abs/1
  Constant4/1 -> Relational Operator1/2
  Abs/1 -> Relational Operator1/1
  Relational Operator1/1 -> TONV_VariableTimeDebounce/1(u)
  Constant1/1 -> TONV_VariableTimeDebounce/3(dT)
  Constant8/1 -> TONV_VariableTimeDebounce/2(T)
  TONV_VariableTimeDebounce/1(y) -> HVSR_flgFrstRsKVld/1, Switch3/2

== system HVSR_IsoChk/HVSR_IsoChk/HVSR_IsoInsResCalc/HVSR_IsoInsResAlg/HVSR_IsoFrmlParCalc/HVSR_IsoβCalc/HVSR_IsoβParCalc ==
  HVSR_uScndRsVlot : Inport
  BSPR_uBattVolt : Inport  Port=2
  Trigger : TriggerPort  VariantControl=Variant  PortDimensions=1
  Add : Sum  Inputs=+-
  Compare To Zero : simulink/Logic and Bit Operations/Compare To Zero  relop=>  OutDataTypeStr=boolean
  Divide : Product  Inputs=*/
  Switch : Switch  Criteria=u2 ~= 0
  HVSR_numIsoScndVal : Outport
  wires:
  BSPR_uBattVolt/1 -> Add/1, Switch/3
  Add/1 -> Divide/1
  Divide/1 -> HVSR_numIsoScndVal/1
  Switch/1 -> Divide/2
  Compare To Zero/1 -> Switch/2
  HVSR_uScndRsVlot/1 -> Add/2, Switch/1, Compare To Zero/1

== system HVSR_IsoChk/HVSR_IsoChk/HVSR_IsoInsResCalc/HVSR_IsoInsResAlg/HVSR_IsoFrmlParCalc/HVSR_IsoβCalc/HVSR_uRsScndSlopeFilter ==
  HVSR_uIsoRsVolt : Inport  OutDataTypeStr=single
  HVSR_kSlopeVal : Inport  Port=2
  HVSR_tiIsoChkCycl_T : Inport  Port=3
  HVSR_numSlopeCnfrm : Inport  Port=4
  Chart : Stateflow chart  TreatAsAtomicUnit=on
  HVSR_bSlopeVld : Outport  OutDataTypeStr=boolean
  ISOFilterSta : Outport  Port=2  OutDataTypeStr=uint8
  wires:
  HVSR_numSlopeCnfrm/1 -> Chart/4(HVSR_numSlopeCnfrm)
  HVSR_tiIsoChkCycl_T/1 -> Chart/3(HVSR_tiIsoChkCycl_T)
  Chart/2(ISOFilterSta) -> ISOFilterSta/1
  HVSR_kSlopeVal/1 -> Chart/2(HVSR_kSlopeVal)
  Chart/1(HVSR_bSlopeVld) -> HVSR_bSlopeVld/1
  HVSR_uIsoRsVolt/1 -> Chart/1(HVSR_uIsoRsVolt)

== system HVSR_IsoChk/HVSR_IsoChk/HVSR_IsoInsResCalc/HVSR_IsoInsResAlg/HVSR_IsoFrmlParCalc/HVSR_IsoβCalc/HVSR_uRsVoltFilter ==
  HVSR_uIsoRsVolt : Inport  OutDataTypeStr=single
  Abs : Abs
  Constant1 : Constant  Value=HVSR_tiTaskTime_C  OutDataTypeStr=single
  Constant2 : Constant  Value=HVSR_cofPosVoltfilter_C  OutDataTypeStr=single
  Constant3 : Constant  Value=0  OutDataTypeStr=single
  Constant4 : Constant  Value=HVSR_uIsoKVoltThres_C  OutDataTypeStr=single
  Constant8 : Constant  Value=HVSR_tiChkFilteTime_C  OutDataTypeStr=single
  K_Lowpass : Subsystem  TreatAsAtomicUnit=on  RTWFcnName=K_Lowpass  RTWFileName=SrvLib
  Relational Operator1 : RelationalOperator  Operator=<=  OutDataTypeStr=boolean  RndMeth=Simplest
  Subtract : Sum  Inputs=+-
  Switch3 : Switch  Criteria=u2 ~= 0
  TONV_VariableTimeDebounce : Subsystem  TreatAsAtomicUnit=on  RTWFcnName=TONV_VariableTimeDebounce  RTWFileName=SrvLib
  HVSR_uIsoScndRsVolt : Outport
  HVSR_uScndRsVlot : Outport  Port=2
  HVSR_flgScndRsKVld : Outport  Port=3
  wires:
  Switch3/1 -> HVSR_uScndRsVlot/1
  HVSR_uIsoRsVolt/1 -> Subtract/2, Switch3/1, HVSR_uIsoScndRsVolt/1, K_Lowpass/2(u)
  Constant3/1 -> Switch3/3
  Constant2/1 -> K_Lowpass/1(k)
  K_Lowpass/1(y) -> Subtract/1
  Subtract/1 -> Abs/1
  Constant4/1 -> Relational Operator1/2
  Abs/1 -> Relational Operator1/1
  Relational Operator1/1 -> TONV_VariableTimeDebounce/1(u)
  Constant1/1 -> TONV_VariableTimeDebounce/3(dT)
  Constant8/1 -> TONV_VariableTimeDebounce/2(T)
  TONV_VariableTimeDebounce/1(y) -> HVSR_flgScndRsKVld/1, Switch3/2

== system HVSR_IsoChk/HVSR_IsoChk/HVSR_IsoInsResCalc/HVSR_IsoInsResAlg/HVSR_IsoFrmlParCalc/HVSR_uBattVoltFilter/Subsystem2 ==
  In1 : Inport
  Constant : Constant  Value=3  OutDataTypeStr=single
  Constant1 : Constant  Value=3  OutDataTypeStr=single
  Delay : Delay  DelayLength=1  InitialCondition=0
  Delay1 : Delay  InitialCondition=0
  Delay2 : Delay  DelayLength=3  InitialCondition=0
  Delay6 : Delay  DelayLength=4  InitialCondition=0
  Delay7 : Delay  DelayLength=5  InitialCondition=0
  Divide : Product  Inputs=*/
  Divide1 : Product  Inputs=*/
  Sum{,1..2,8} (4 alike) : Sum  Inputs=|++
  Sum3 : Sum  Inputs=|+-
  Out1 : Outport
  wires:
  Constant1/1 -> Divide1/2
  Sum8/1 -> Divide1/1
  Delay7/1 -> Sum8/2
  Sum2/1 -> Sum8/1
  Delay6/1 -> Sum2/2
  Delay2/1 -> Sum2/1
  Divide1/1 -> Sum3/2
  Divide/1 -> Sum3/1
  Constant/1 -> Divide/2
  Sum1/1 -> Divide/1
  Sum/1 -> Sum1/2
  Delay1/1 -> Sum/2
  Delay/1 -> Sum/1
  In1/1 -> Delay1/1, Delay2/1, Delay6/1, Delay7/1, Delay/1, Sum1/1
  Sum3/1 -> Out1/1

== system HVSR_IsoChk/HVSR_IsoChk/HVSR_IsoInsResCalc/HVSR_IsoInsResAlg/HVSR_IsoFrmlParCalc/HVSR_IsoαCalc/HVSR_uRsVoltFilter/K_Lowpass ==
  k : Inport
  u : Inport  Port=2
  Add : Sum
  Constant2 : Constant  Value=0  OutDataTypeStr=boolean
  Delay : Delay  DelayLength=1  InitialCondition=1
  Product : Product
  Subtract : Sum  Inputs=+-
  Switch1 : Switch  Criteria=u2 > Threshold
  Unit Delay : UnitDelay  SampleTime=-1
  y : Outport
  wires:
  u/1 -> Subtract/1, Switch1/1
  Switch1/1 -> Unit Delay/1, y/1
  Delay/1 -> Switch1/2
  Add/1 -> Switch1/3
  Subtract/1 -> Product/2
  Unit Delay/1 -> Add/2, Subtract/2
  Constant2/1 -> Delay/1
  Product/1 -> Add/1
  k/1 -> Product/1

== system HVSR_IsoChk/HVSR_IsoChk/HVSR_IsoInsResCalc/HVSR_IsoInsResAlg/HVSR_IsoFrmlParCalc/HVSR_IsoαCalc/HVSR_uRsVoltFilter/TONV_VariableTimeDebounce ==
  note: Turn On Delay Time Deboune
  u : Inport
  T : Inport  Port=2
  dT : Inport  Port=3
  Add : Sum
  Constant1 : Constant  Value=0  OutDataTypeStr=single
  Constant2 : Constant  OutDataTypeStr=uint8
  Constant3 : Constant  Value=0  OutDataTypeStr=uint8
  Delay : Delay  DelayLength=1  InitialCondition=0
  MinMax : MinMax  Inputs=2
  Product : Product  OutMin=[0]  OutMax=[65535]  OutDataTypeStr=single
  Relational Operator : RelationalOperator  Operator=>  OutDataTypeStr=boolean  RndMeth=Simplest
  Switch : Switch  Criteria=u2 ~= 0
  Switch1 : Switch  Criteria=u2 ~= 0
  y : Outport
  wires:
  Switch1/1 -> Product/1
  Constant3/1 -> Switch1/3
  Constant2/1 -> Switch1/1
  u/1 -> Switch1/2, Switch/2
  dT/1 -> Switch/1
  Constant1/1 -> Switch/3
  Add/1 -> Product/2
  Product/1 -> Relational Operator/1, Delay/1
  Switch/1 -> Add/1
  Delay/1 -> MinMax/2
  Relational Operator/1 -> y/1
  T/1 -> MinMax/1, Relational Operator/2
  MinMax/1 -> Add/2

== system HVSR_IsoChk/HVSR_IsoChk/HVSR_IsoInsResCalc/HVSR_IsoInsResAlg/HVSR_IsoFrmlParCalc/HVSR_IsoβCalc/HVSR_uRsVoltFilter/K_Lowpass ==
  k : Inport
  u : Inport  Port=2
  Add : Sum
  Constant2 : Constant  Value=0  OutDataTypeStr=boolean
  Delay : Delay  DelayLength=1  InitialCondition=1
  Product : Product
  Subtract : Sum  Inputs=+-
  Switch1 : Switch  Criteria=u2 > Threshold
  Unit Delay : UnitDelay  SampleTime=-1
  y : Outport
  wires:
  u/1 -> Subtract/1, Switch1/1
  Switch1/1 -> Unit Delay/1, y/1
  Delay/1 -> Switch1/2
  Add/1 -> Switch1/3
  Subtract/1 -> Product/2
  Unit Delay/1 -> Add/2, Subtract/2
  Constant2/1 -> Delay/1
  Product/1 -> Add/1
  k/1 -> Product/1

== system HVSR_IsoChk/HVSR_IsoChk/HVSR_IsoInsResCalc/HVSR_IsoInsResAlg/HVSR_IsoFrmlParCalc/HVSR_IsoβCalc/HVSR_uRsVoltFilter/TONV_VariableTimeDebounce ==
  note: Turn On Delay Time Deboune
  u : Inport
  T : Inport  Port=2
  dT : Inport  Port=3
  Add : Sum
  Constant1 : Constant  Value=0  OutDataTypeStr=single
  Constant2 : Constant  OutDataTypeStr=uint8
  Constant3 : Constant  Value=0  OutDataTypeStr=uint8
  Delay : Delay  DelayLength=1  InitialCondition=0
  MinMax : MinMax  Inputs=2
  Product : Product  OutMin=[0]  OutMax=[65535]  OutDataTypeStr=single
  Relational Operator : RelationalOperator  Operator=>  RndMeth=Simplest
  Switch : Switch  Criteria=u2 ~= 0
  Switch1 : Switch  Criteria=u2 ~= 0
  y : Outport
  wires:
  Switch1/1 -> Product/1
  Constant3/1 -> Switch1/3
  Constant2/1 -> Switch1/1
  u/1 -> Switch1/2, Switch/2
  dT/1 -> Switch/1
  Constant1/1 -> Switch/3
  Add/1 -> Product/2
  Product/1 -> Relational Operator/1, Delay/1
  Switch/1 -> Add/1
  Delay/1 -> MinMax/2
  Relational Operator/1 -> y/1
  T/1 -> MinMax/1, Relational Operator/2
  MinMax/1 -> Add/2

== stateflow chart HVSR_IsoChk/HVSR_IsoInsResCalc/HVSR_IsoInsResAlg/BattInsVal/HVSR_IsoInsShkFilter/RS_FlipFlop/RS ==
  state RS_FlipFlop
    (default) -> (junction 3)
    (junction 3) -> (junction 5) : [R]
    (junction 3) -> (junction 12)
    (junction 5) -> (junction 7) : {Q=boolean(0);nQ=boolean(1);}
    (junction 12) -> (junction 14) : [S]
    (junction 14) -> (junction 16) : {Q=boolean(1);nQ=boolean(0);}
    (junction 12) -> (junction 18)
    (junction 16) -> (junction 18)
    (junction 7) -> (junction 18)
    (junction 18) -> (junction 21)
  (default) -> RS_FlipFlop
  (junction 24) -> RS_FlipFlop
  (junction 25) -> (junction 24)
  RS_FlipFlop -> (junction 23)
  (junction 23) -> (junction 25)
  data: S input boolean; R input boolean; Q output boolean; nQ output boolean
